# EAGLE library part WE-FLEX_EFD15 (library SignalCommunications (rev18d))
WE-FLEX Flexible Transformer for DC/DC Converter Characteristics Transformer with 6 identical windings 4 sizes with 5 different lengths of air gap each Insulation test voltage 500 VAC Low leakage inductance Operating temperature: –40 ºC to +125 ºC By using different circuits more than 375 transformer solutions and about 125 choke solutions possible. Consequently, quick prototyping possibilities Applications All kind of switching regulators -Flyback converters -Forward converters -Push-pull converters -Step-up/step-down converters -SEPIC converter Details see: http://katalog.we-online.de/en/pbs/WE-FLEX? Updated by Dan Xu 2014-07-07 2014 (C) Wurth Elektronik
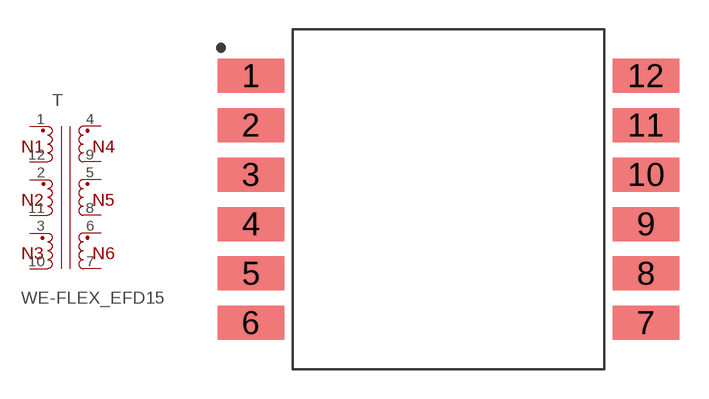
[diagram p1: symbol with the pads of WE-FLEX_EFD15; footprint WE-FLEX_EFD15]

Designator prefix T

## WE-FLEX_EFD15_749196301, WE-FLEX_EFD15_749196311, WE-FLEX_EFD15_749196321, WE-FLEX_EFD15_749196331, WE-FLEX_EFD15_749196341  [WE-FLEX_EFD15]
1  1  pas
2  11  pas
3  9  pas
4  2  pas
5  4  pas
6  6  pas
7  7  pas
8  5  pas
9  3  pas
10  8  pas
11  10  pas
12  12  pas

## Footprint WE-FLEX_EFD15 (pad centres in mm)
smd 3.43 x 1.75: 1 -10.155,6.35; 2 -10.155,3.81; 3 -10.155,1.27; 4 -10.155,-1.27; 5 -10.155,-3.81; 6 -10.155,-6.35; 7 10.155,-6.35; 8 10.155,-3.81; 9 10.155,-1.27; 10 10.155,1.27; 11 10.155,3.81; 12 10.155,6.35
